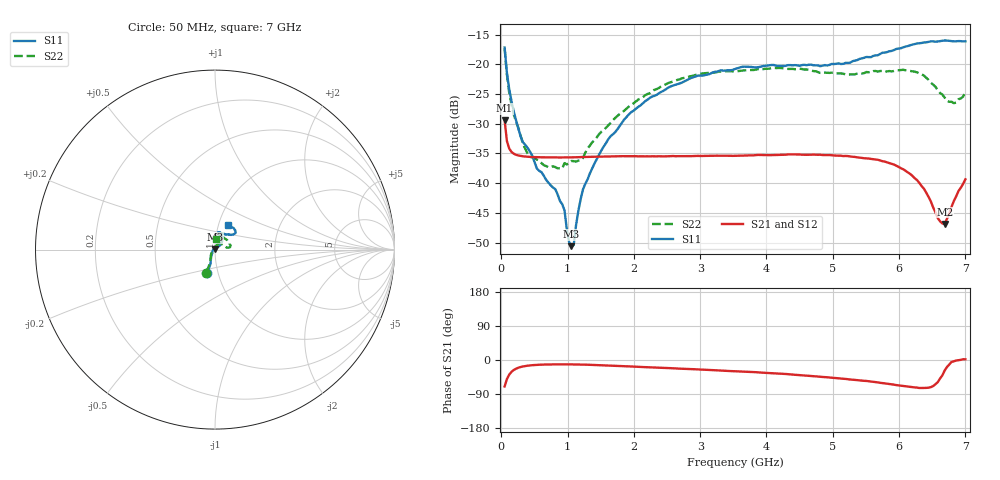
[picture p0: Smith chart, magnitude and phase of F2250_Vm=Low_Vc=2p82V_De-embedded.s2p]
! Integrated Device Technology
! Corporate Headquarters
! 6024 Silver Creek Valley Road
! San Jose, CA 95138  USA
! Phone:  1-408-284-8200
! Toll Free:  1-800-223-1366
! Webpage:  http://www.idt.com/
! Timing and RF Division
! 515 Groton Road, Suite 102
! Westford, MA 01886-6024
! Device:  F2250
! Description: Voltage Variable RF Attenuator
! Frequency:  50.0 -  6000.00 MHz
! Package:  3x3 mm Thin QFN Plastic Package: 16 pin
! Ports:  2 RF, 3 DC
!  Pin  1  = GND
!  Pin  2  = NC
!  Pin  3  = RF1  = Port 1
!  Pin  4  = NC
!  Pin  5  = GND
!  Pin  6  = GND
!  Pin  7  = GND
!  Pin  8  = GND
!  Pin  9  = NC
!  Pin 10  = RF2  = Port 2
!  Pin 11  = NC
!  Pin 12  = GND
!  Pin 13  = GND
!  Pin 14  = VCNTRL
!  Pin 15  = VDD
!  Pin 16  = VMODE
! Vcntrl:  2.820 Volts
! Vmode:  +0.000 Volts
! Vdd:  +3.30  Volts
! Current:  1.175 mA
! Data:  The device was measured on a the F2250 evaluation board which has
!  individual transmission lines to the RF pins.  Data was collected
!  using a calibrated network analyzer.  The evaluation board was
!  de-embedded using a TRL calibration technique.
!  The reference plane is the edge of the package pin.
! Misc:  SN 10
!  Action Tracker AT0258
! Date Measured:  2014-11-26
! Date:  2015-10-15  MJV
! Note:
!  Integrated Device Technology supplies this data as a sample of measured
!  data at the package pin for this product.  Your particular data for this
!  product may vary.
!  Data was taken at 25 degrees C.
!  Integrated Device Technology reserves the right to change this data at anytime.
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# GHz S dB R 50
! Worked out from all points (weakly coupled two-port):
!   201 points, 50 MHz to 7 GHz, reference 50 ohm
!   highest |S21| = -29.41 dB at 50 MHz (marker M1); lowest = -46.9 dB at 6.687 GHz (marker M2)
!   lowest |S11| = -50.6 dB at 1.058 GHz (marker M3), VSWR 1.01, Z = 49.8 + j0.246 ohm
!   |S11| at or under -10 dB: start of sweep to end of sweep
!   |S22| runs from -37.5 to -17.3 dB; largest |S21 - S12| = 7.1e-05
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0.05  -17.18 -108.6  -29.41 -69.8  -29.41 -69.8  -17.28 -111.0
0.08475  -21.45 -107.4  -32.92 -50.3  -32.92 -50.3  -21.75 -110.2
0.15425  -26.23 -116.6  -34.76 -31.1  -34.75 -31.1  -26.82 -122.4
0.29325  -32.22 -127.9  -35.43 -18.5  -35.43 -18.5  -32.09 -137.5
0.3975  -34.09 -141.9  -35.56 -15.0  -35.56 -15.0  -35.05 -160.5
0.91875  -43.54 157.8  -35.68 -11.5  -35.69 -11.5  -37.55 133.6
0.9535  -44.59 170.0  -35.69 -11.5  -35.68 -11.5  -36.63 131.1
1.023  -49.94 143.7  -35.67 -11.6  -35.68 -11.6  -36.61 115.9
1.05775  -50.61 123.2  -35.67 -11.6  -35.67 -11.6  -36.28 110.7
1.0925  -50.42 89.2  -35.66 -11.7  -35.66 -11.7  -36.31 106.1
1.162  -44.70 56.8  -35.64 -11.9  -35.64 -11.9  -36.22 95.4
1.2315  -41.07 44.6  -35.61 -12.1  -35.61 -12.1  -35.79 85.9
1.6485  -32.11 42.0  -35.52 -14.6  -35.52 -14.7  -29.87 64.6
1.96125  -28.05 42.2  -35.46 -17.2  -35.46 -17.2  -26.81 56.8
2.37825  -24.87 47.3  -35.48 -20.3  -35.48 -20.3  -23.99 56.8
3.525  -20.79 72.5  -35.40 -29.5  -35.40 -29.6  -21.19 74.7
4.7065  -20.17 72.3  -35.20 -42.6  -35.20 -42.6  -21.14 72.3
5.85325  -17.81 40.5  -36.63 -63.4  -36.63 -63.4  -21.14 23.0
6.27025  -16.51 40.0  -39.49 -72.8  -39.50 -72.8  -21.36 9.7
6.68725  -15.99 48.8  -46.89 -27.8  -46.86 -27.4  -25.63 28.6
6.861  -16.13 55.1  -42.22 -1.4  -42.14 -1.3  -26.46 58.0
7  -16.13 63.2  -39.36 1.9  -39.33 1.7  -24.63 83.1
